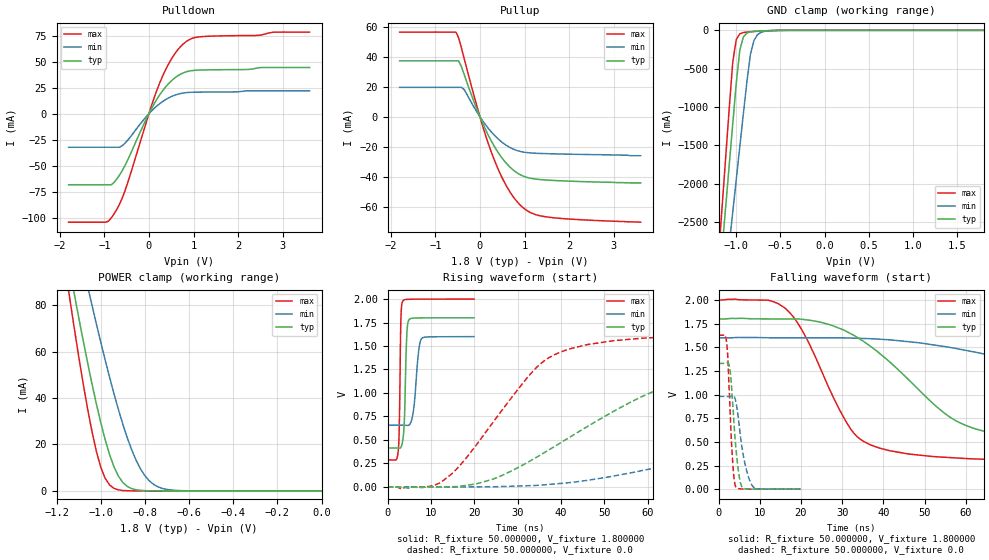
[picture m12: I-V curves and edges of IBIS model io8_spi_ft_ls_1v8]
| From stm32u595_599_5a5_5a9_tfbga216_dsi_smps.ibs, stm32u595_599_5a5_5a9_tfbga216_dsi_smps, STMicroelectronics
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|   Model io8_spi_ft_ls_1v8
[Model]  io8_spi_ft_ls_1v8
Model_type I/O
Polarity   Non-Inverting
Enable   Active-Low
Vinl =   0.540000V
Vinh =   1.260000V
Vmeas =  0.900000V
Cref =   50.000000pF
Rref =   100.000000M
Vref =   0.0V
C_comp   3.338500pF   3.332300pF   3.378900pF
[Temperature Range]   25.000000   0.140000k   -40.000000
[Pullup Reference]   1.800000V   1.600000V   2.000000V
[Pulldown Reference]   0.0V   0.0V   0.0V
[POWER Clamp Reference]   1.800000V   1.600000V   2.000000V
[GND Clamp Reference]   0.0V   0.0V   0.0V
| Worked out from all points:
|   slope of the pulldown table from 0 to 0.27 V, typ, clamps not added: 13.6 ohm
|   slope of the pullup table from 0 to 0.27 V, typ, clamps not added: 15.9 ohm
|   GND clamp passes 1 mA (typ) near -0.51 V on its own axis
|   POWER clamp passes 1 mA (typ) near -0.86 V on its own axis
|   rising waveform, R_fixture 50.000000, V_fixture 1.800000: 20-80 % time 490ps typ, 1.02ns min, 317ps max; typ from 0.414 V to 1.8 V
|   rising waveform, R_fixture 50.000000, V_fixture 0.0: 20-80 % time 31.5ns typ, 69.2ns min, 16.6ns max; typ from 0 V to 1.33 V
|   falling waveform, R_fixture 50.000000, V_fixture 1.800000: 20-80 % time 22.7ns typ, 57.7ns min, 11.6ns max; typ from 1.8 V to 0.414 V
|   falling waveform, R_fixture 50.000000, V_fixture 0.0: 20-80 % time 1.43ns typ, 2.11ns min, 1.03ns max; typ from 1.33 V to 0 V
[Pulldown]
|Voltage   I(typ)   I(min)   I(max)
-1.8V     -68.38mA   -32.32mA   -104.4mA
-960mV    -68.38mA   -32.32mA   -104.4mA
-780mV    -66.07mA   -32.32mA   -96.42mA
-660mV    -59.2mA    -32.31mA   -87.22mA
-540mV    -50.22mA   -28.51mA   -74.66mA
0V        0A         -300fA     0A
240mV     18.04mA    9.599mA    29.42mA
480mV     30.68mA    16.02mA    50.95mA
780mV     39.47mA    19.98mA    67.56mA
960mV     41.44mA    20.62mA    72.37mA
1.14V     41.99mA    20.78mA    74.01mA
3.6V      44.44mA    22.06mA    78.55mA
[Pullup]
|Voltage   I(typ)   I(min)   I(max)
-1.8V     37.47mA    19.74mA    56.73mA
-540mV    37.47mA    19.74mA    56.73mA
-480mV    37.47mA    19.74mA    53.05mA
-360mV    28.94mA    18.47mA    39.74mA
0V        630fA      250pA      10fA
300mV     -18.63mA   -11.6mA    -27.18mA
600mV     -31.41mA   -19.24mA   -46.67mA
780mV     -36.41mA   -22mA      -54.88mA
960mV     -39.54mA   -23.52mA   -60.64mA
1.2V      -41.44mA   -24.28mA   -64.94mA
1.56V     -42.42mA   -24.69mA   -67.24mA
3.6V      -44.2mA    -26mA      -70.5mA
[GND_clamp]
|Voltage   I(typ)   I(min)   I(max)
-1.8V     -9.908A    -9.683A    -9.994A
-1.2V     -3.383A    -4.084A    -2.934A
-1.16V    -2.841A    -3.655A    -2.294A
-1.12V    -2.299A    -3.226A    -1.656A
-1.04V    -1.218A    -2.369A    -414.2mA
-1V       -684.7mA   -1.941A    -119.2mA
-960mV    -257.2mA   -1.514A    -45.66mA
-920mV    -87.03mA   -1.089A    -28.93mA
-840mV    -19.35mA   -312.8mA   -18.96mA
-800mV    -13.55mA   -132.4mA   -15.49mA
-720mV    -8.042mA   -25.66mA   -9.49mA
1.8V      0A         13.64nA    0A
[POWER_clamp]
|Voltage   I(typ)   I(min)   I(max)
-1.8V     470.8mA    433.7mA    554.6mA
-1.14V    95.25mA    122.7mA    82.82mA
-1.12V    84.97mA    114mA      70.27mA
-1.06V    55.51mA    88.42mA    35.67mA
-1.04V    46.34mA    80.15mA    25.76mA
-1V       29.51mA    64.13mA    10.3mA
-940mV    10.39mA    41.86mA    1.109mA
-900mV    3.624mA    28.77mA    182.8uA
-840mV    490.7uA    13.24mA    11.35uA
-800mV    116.8uA    6.532mA    1.77uA
-740mV    13.2uA     1.724mA    109.3nA
0V        0A         18.75nA    0A
[Ramp]
| variable   typ   min   max
dV/dt_r  0.79770/31.44026n   0.58790/69.07996n   0.97668/16.60961n
dV/dt_f  0.83162/22.59984n   0.56509/57.64081n   1.02769/11.60568n
R_load = 50.000000
[Rising Waveform]
R_fixture= 50.000000
V_fixture= 1.800000
V_fixture_min= 1.600000
V_fixture_max= 2.000000
|time   V(typ)   V(min)   V(max)
0s        414mV      656.9mV    287.2mV
2.482ns   413.4mV    656.9mV    390.6mV
2.723ns   412.4mV    657mV      688mV
3.083ns   422.5mV    657mV      1.796V
3.483ns   489.7mV    656.9mV    1.976V
3.884ns   717.1mV    656.7mV    1.992V
4.444ns   1.624V     655mV      1.996V
4.925ns   1.778V     656.8mV    1.997V
7.808ns   1.799V     1.576V     1.999V
19.94ns   1.8V       1.6V       2V
[Rising Waveform]
R_fixture= 50.000000
V_fixture= 0.0
V_fixture_min= 0.0
V_fixture_max= 0.0
|time   V(typ)   V(min)   V(max)
0s        1.85nV     146.7nV    1.205nV
12.01ns   -336.4uV   -211.4uV   40.95mV
24.02ns   78.48mV    897.4uV    668.2mV
35.24ns   338.8mV    18.38mV    1.308V
52.85ns   822.1mV    121mV      1.56V
65.67ns   1.09V      239.1mV    1.599V
81.68ns   1.226V     398.9mV    1.618V
122.5ns   1.31V      739.6mV    1.627V
154.6ns   1.324V     876.2mV    1.628V
398.8ns   1.33V      980.3mV    1.628V
[Falling Waveform]
R_fixture= 50.000000
V_fixture= 1.800000
V_fixture_min= 1.600000
V_fixture_max= 2.000000
|time   V(typ)   V(min)   V(max)
0s        1.8V       1.6V       2V
16.02ns   1.8V       1.6V       1.918V
20.82ns   1.793V     1.6V       1.637V
33.63ns   1.606V     1.596V     555.8mV
52.05ns   906mV      1.526V     344.9mV
61.66ns   647.7mV    1.454V     320.3mV
76.88ns   524.8mV    1.294V     302.7mV
109.7ns   449.5mV    926.7mV    290.5mV
144.9ns   426.1mV    773.4mV    287.9mV
398.8ns   414mV      656.9mV    287.2mV
[Falling Waveform]
R_fixture= 50.000000
V_fixture= 0.0
V_fixture_min= 0.0
V_fixture_max= 0.0
|time   V(typ)   V(min)   V(max)
0s        1.33V      980.3mV    1.628V
1.562ns   1.329V     980.3mV    1.631V
2.002ns   1.333V     980.3mV    1.531V
2.763ns   1.257V     980.2mV    856mV
3.323ns   964.9mV    986.7mV    350.7mV
4.164ns   451.3mV    928.9mV    25.88mV
5.526ns   36.37mV    484.6mV    2.352mV
6.727ns   3.194mV    209.3mV    914.9uV
8.368ns   891.7uV    25.99mV    419.4uV
19.94ns   1.85nV     146.7nV    1.205nV
